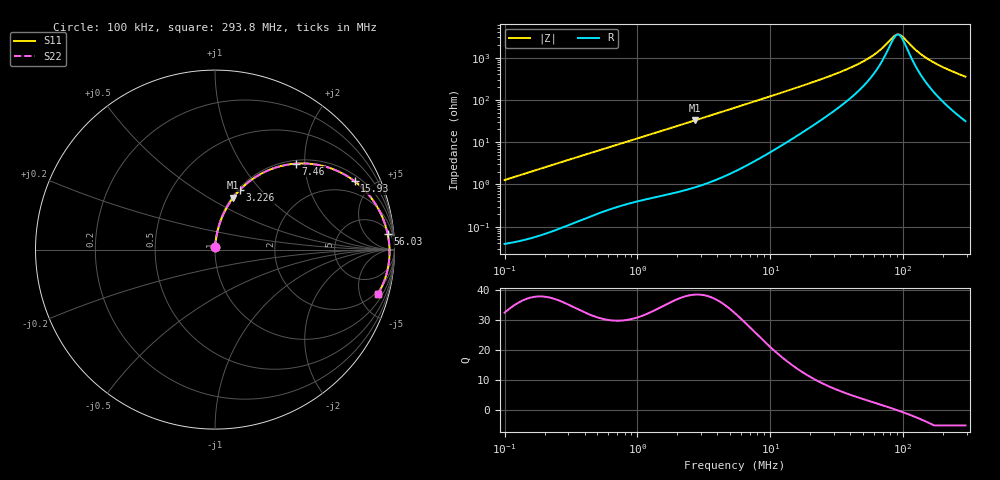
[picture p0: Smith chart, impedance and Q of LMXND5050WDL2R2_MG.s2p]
! LMXND5050WDL2R2_MG  S-PARAMETER MODEL  ( General Type )
! Model Generated by TAIYO YUDEN Corporation (http://www.ty-top.com)
! Version 1.0
! TAIYO YUDEN Control No. 191023NI43SB-FBB
! Copyright(c) 2019 TAIYO YUDEN CO.,LTD. All Rights Reserved.
! Product Description (link to TY-COMPAS)
! https://ds.yuden.co.jp/TYCOMPAS/or/detail?pn=LMXND5050WDL2R2NMG&u=M
! Products Name : Inductors
! Characteristics :
!  Inductance : 2.2 uH , SRF(min) : 51 MHz , DC Resistance(max) : 0.0348 Ohm
!  Rated Current : Saturation :4100 mA , Temp Rise : 3100 mA
!  Case Size : 4.9 x 4.9 / 0.193 x 0.193 [mm/inch] , Thickness : 2.4 / 0.094 [mm/inch]
!  (Conditions: Temperature = 25 degC , DC Bias Current/Voltage = 0A / 0V)
! External Node Assignments :
!  1  o---GGG---o  2
! GND o---------o GND
! Frequency Range : 0.1MHz  -  293.796821MHz  [ 402 STEP ]
# MHz S RI R 50
! Freq[MHz].  S11 Real  S11 Imag  S21 Real  S21 Imag  S12 Real  S12 Imag  S22 Real  S22 Imag
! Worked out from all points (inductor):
!   401 points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, 100 kHz to 293.8 MHz, reference 50 ohm
!   read as one part in series: L = 2.02 uH near 104.1 kHz
!   highest Q = 38.4 at 2.695 MHz (marker M1), where L = 1.92 uH
!   self-resonance near 91.14 MHz
!   S11 on the Smith chart (normalised r, x): 100 kHz: 1.00, +0.03; 3.226 MHz: 1.02, +0.78; 7.46 MHz: 1.07, +1.80; 15.93 MHz: 1.28, +3.92; 56.03 MHz: 7, +19; 293.8 MHz: 1.63, -7.06
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0.1  0.000551 0.0127  0.9994 -0.0127  0.9994 -0.0127  0.000551 0.0127
0.380976  0.00371 0.0475  0.9963 -0.0475  0.9963 -0.0475  0.00371 0.0475
0.797429  0.0127 0.0966  0.9873 -0.0966  0.9873 -0.0966  0.0127 0.0966
1.451429  0.0349 0.1693  0.9651 -0.1693  0.9651 -0.1693  0.0349 0.1693
2.695066  0.1018 0.2897  0.8982 -0.2897  0.8982 -0.2897  0.1018 0.2897
3.225526  0.1379 0.3319  0.8621 -0.3319  0.8621 -0.3319  0.1379 0.3319
5.420303  0.3051 0.4452  0.6949 -0.4452  0.6949 -0.4452  0.3051 0.4452
7.460113  0.4505 0.479  0.5495 -0.479  0.5495 -0.479  0.4505 0.479
10.4746  0.613 0.4629  0.387 -0.4629  0.387 -0.4629  0.613 0.4629
15.92979  0.7779 0.3811  0.2221 -0.3811  0.2221 -0.3811  0.7779 0.3811
20.65007  0.8487 0.3148  0.1513 -0.3148  0.1513 -0.3148  0.8487 0.3148
36.84299  0.9355 0.1735  0.0645 -0.1735  0.0645 -0.1735  0.9355 0.1735
56.03086  0.9617 0.0884  0.0383 -0.0884  0.0383 -0.0884  0.9617 0.0884
67.0592  0.9677 0.0551  0.0323 -0.0551  0.0323 -0.0551  0.9677 0.0551
78.67184  0.971 0.0263  0.029 -0.0263  0.029 -0.0263  0.971 0.0263
86.93005  0.9722 0.00847  0.0278 -0.00847  0.0278 -0.00847  0.9722 0.00847
94.15652  0.9726 -0.00587  0.0274 0.00587  0.0274 0.00587  0.9726 -0.00587
99.96794  0.9726 -0.0167  0.0274 0.0167  0.0274 0.0167  0.9726 -0.0167
127.0288  0.97 -0.0611  0.03 0.0611  0.03 0.0611  0.97 -0.0611
155.097  0.9641 -0.1005  0.0359 0.1005  0.0359 0.1005  0.9641 -0.1005
209.245  0.9463 -0.1653  0.0537 0.1653  0.0537 0.1653  0.9463 -0.1653
293.7968  0.9074 -0.2489  0.0926 0.2489  0.0926 0.2489  0.9074 -0.2489
